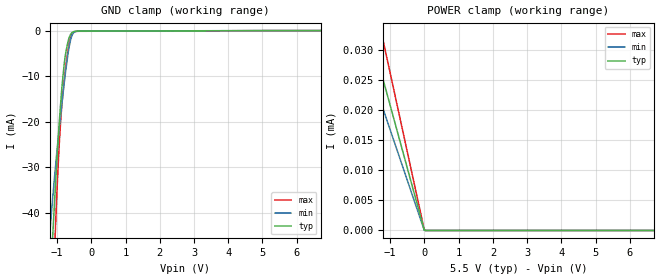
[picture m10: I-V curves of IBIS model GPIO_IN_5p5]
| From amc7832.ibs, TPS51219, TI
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|   Model
[Model]   GPIO_IN_5p5
Model_type   Input
Vinl = 1.65
Vinh = 3.85
|   typ   min   max
C_comp   1pF   1pF   1pF
[Voltage Range]   5.5   5.49   5.51
[Temperature Range]   27   125   -40
[Power Clamp Reference]   5.5   5.49   5.51
[GND Clamp Reference]   -0   -0   -0
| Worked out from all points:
|   GND clamp passes 1 mA (typ) near -0.62 V on its own axis
[GND Clamp]
|   Voltage   I(typ)   I(min)   I(max)
-5.5V     -817.2mA   -581.7mA   -1.063A
-1.21V    -56.99mA   -44.06mA   -76.21mA
-1.127V   -44.92mA   -36.61mA   -58.94mA
-1.078V   -37.98mA   -32.35mA   -49mA
-1.012V   -29.2mA    -26.99mA   -36.62mA
-913mV    -17.59mA   -19.72mA   -21.83mA
-863.5mV  -12.83mA   -16.29mA   -16.55mA
-797.5mV  -7.656mA   -11.87mA   -11.23mA
-748mV    -4.86mA    -8.761mA   -7.96mA
-649mV    -1.572mA   -3.618mA   -2.829mA
-517mV    -226.6uA   -469.4uA   -306.5uA
10.98V    0A         0A         0A
[POWER Clamp]
|   Voltage   I(typ)   I(min)   I(max)
-5.5V     114.6uA    1.467mA    144uA
-4.559V   94.91uA    76.62uA    119.4uA
-1.375V   28.58uA    23.02uA    35.96uA
-1.144V   23.77uA    19.14uA    29.91uA
-5.5mV    56.77nA    24.08nA    97.36nA
10.98V    0A         0A         0A
